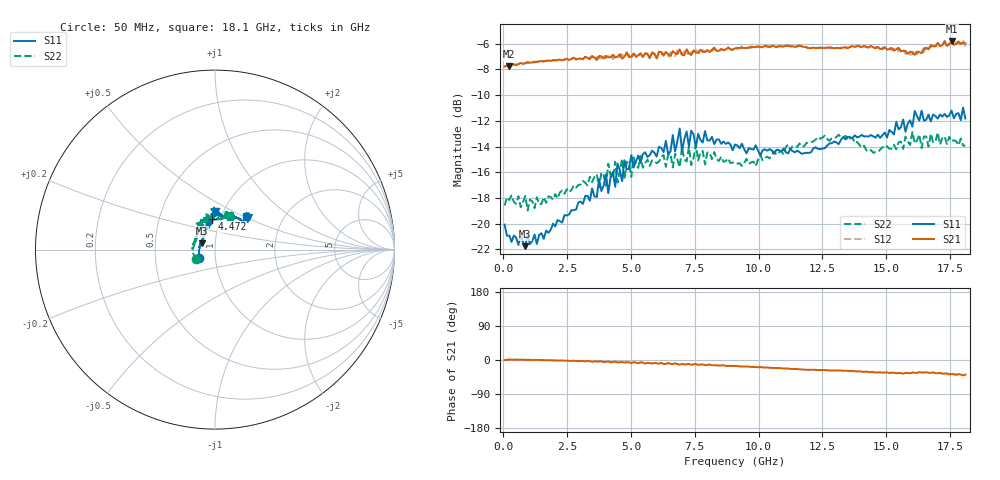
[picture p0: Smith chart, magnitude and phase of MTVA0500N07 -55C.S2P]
! Network Analyzer HP8720D.06.14 Serial No. US36140669
!  5 Jul 2005  08:48:17
! Frequency  S11  S21  S12  S22
# HZ  S  DB R 50
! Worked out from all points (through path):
!   201 points, 50 MHz to 18.1 GHz, reference 50 ohm
!   highest |S21| = -5.80 dB at 17.56 GHz (marker M1); lowest = -7.8 dB at 230.5 MHz (marker M2)
!   group delay of S21, straight-line fit = 6.63 ps
!   lowest |S11| = -21.8 dB at 862.2 MHz (marker M3), VSWR 1.18, Z = 43 + j3.07 ohm
!   |S11| at or under -10 dB: start of sweep to end of sweep
!   |S22| runs from -19.0 to -12.9 dB; largest |S21 - S12| = 0.024
!   S11 on the Smith chart (normalised r, x): 50 MHz: 0.84, -0.08; 4.472 GHz: 0.91, +0.32; 18.1 GHz: 1.31, +0.52
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5e7  -20.08 -152.6  -7.76 -0.2  -7.78 -0.1  -18.59 -152.2
2.305e8  -20.93 -177.6  -7.76 1.3  -7.80 1.3  -18.17 179.5
8.6225e8  -21.76 154.3  -7.52 0.4  -7.46 0.7  -17.86 166.2
3.1185e9  -18.47 114.7  -7.20 -2.9  -7.21 -3.4  -16.67 133.3
4.021e9  -16.16 106.5  -6.94 -4.9  -7.12 -4.0  -17.05 124.7
4.11125e9  -17.63 105.1  -7.04 -3.7  -6.97 -5.6  -15.33 123.2
4.382e9  -17.14 101.7  -7.06 -4.2  -6.93 -5.9  -15.19 123.4
4.47225e9  -15.32 96.2  -7.01 -6.4  -6.96 -4.4  -16.81 126.8
4.65275e9  -16.70 95.9  -7.15 -5.1  -6.83 -5.9  -14.97 125.0
4.743e9  -15.07 98.5  -7.00 -6.6  -7.05 -5.4  -16.57 120.6
5.104e9  -15.64 99.8  -6.76 -5.9  -6.76 -7.2  -14.85 115.3
6.09675e9  -14.02 91.9  -6.65 -9.3  -6.59 -8.9  -15.17 110.5
6.7285e9  -14.38 95.1  -6.72 -8.3  -6.95 -10.1  -14.56 103.0
6.909e9  -12.59 91.5  -6.44 -12.0  -6.70 -10.3  -15.60 101.3
6.99925e9  -14.35 91.1  -6.84 -10.1  -6.85 -12.4  -14.06 101.9
7.36025e9  -12.76 83.9  -6.88 -12.6  -6.66 -10.8  -15.43 105.6
7.54075e9  -14.09 85.1  -6.68 -10.5  -6.45 -13.0  -13.85 104.0
9.075e9  -13.84 86.4  -6.35 -15.9  -6.32 -15.9  -15.24 89.6
1.21435e10  -14.15 65.4  -6.30 -25.7  -6.25 -25.8  -13.61 73.8
1.512175e10  -12.71 42.6  -6.42 -34.3  -6.24 -33.7  -14.17 69.7
1.75585e10  -11.20 47.5  -5.80 -37.2  -5.84 -37.0  -13.61 68.4
1.81e10  -11.82 46.9  -5.97 -38.7  -6.21 -39.7  -13.92 65.1
